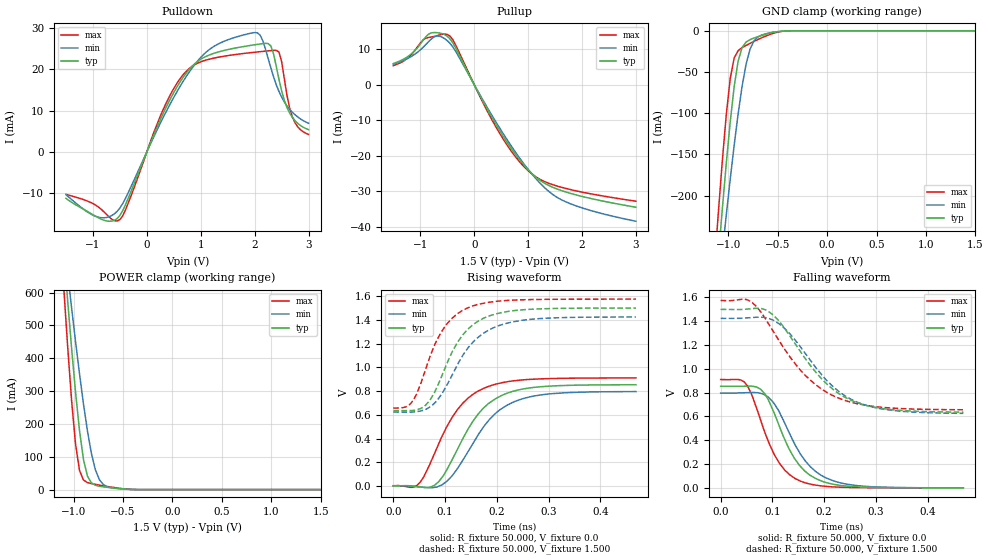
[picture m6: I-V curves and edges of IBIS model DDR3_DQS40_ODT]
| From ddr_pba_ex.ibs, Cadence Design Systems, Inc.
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|   Model DDR3_DQS40_ODT
[Model]   DDR3_DQS40_ODT
Model_type I/O
Polarity   Non-Inverting
Enable   Active-High
Vinl   =   0.703V
Vinh   =   0.796V
C_comp   1.640pF   1.630pF   1.688pF
C_comp_pullup   0.471pF   0.511pF   0.476pF
C_comp_pulldown 1.168pF   1.119pF   1.211pF
[Model Spec]
Vinh   0.796V   NA   NA
Vinl   0.703V   NA   NA
Vmeas   0.750V   NA   NA
[Add Submodel]
|  Submodel_name   Mode
DDR3_DQS_ODT60   Non-Driving
[Temperature Range]   27.000   0.125k   -40.000
[Voltage Range]   1.500V   1.425V   1.575V
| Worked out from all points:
|   slope of the pulldown table from 0 to 0.225 V, typ, clamps not added: 31.8 ohm
|   slope of the pullup table from 0 to 0.225 V, typ, clamps not added: 34.8 ohm
|   GND clamp passes 1 mA (typ) near -0.50 V on its own axis
|   POWER clamp passes 1 mA (typ) near -0.45 V on its own axis
|   rising waveform, R_fixture 50.000, V_fixture 0.0: 20-80 % time 73ps typ, 78.2ps min, 70.9ps max; typ from 0 V to 0.853 V
|   rising waveform, R_fixture 50.000, V_fixture 1.500: 20-80 % time 63.7ps typ, 72.4ps min, 57.6ps max; typ from 0.635 V to 1.5 V
|   falling waveform, R_fixture 50.000, V_fixture 0.0: 20-80 % time 58.1ps typ, 64.5ps min, 53.2ps max; typ from 0.854 V to 0 V
|   falling waveform, R_fixture 50.000, V_fixture 1.500: 20-80 % time 97.1ps typ, 96.2ps min, 101ps max; typ from 1.5 V to 0.636 V
[Pulldown]
|Voltage   I(typ)   I(min)   I(max)
-1.5V     -11.24mA   -10.36mA   -10.27mA
-900mV    -15.94mA   -15.8mA    -13.32mA
-500mV    -15.38mA   -13.58mA   -16.39mA
250mV     7.818mA    6.93mA     8.666mA
600mV     16.62mA    15.5mA     17.43mA
1.1V      23.14mA    24.16mA    22.24mA
1.7V      25.29mA    27.98mA    23.68mA
2.1V      26.12mA    28.29mA    24.27mA
2.3V      25.65mA    20.33mA    24.52mA
2.45V     17.59mA    14.66mA    24.19mA
2.7V      8.354mA    9.586mA    8.44mA
3V        5.378mA    6.93mA     4.234mA
[Pullup]
|Voltage   I(typ)   I(min)   I(max)
-1.5V     5.907mA    5.675mA    5.311mA
-1.2V     8.216mA    7.612mA    7.902mA
-950mV    12.44mA    10.43mA    12.49mA
-800mV    14.52mA    12.76mA    13.36mA
-650mV    14.53mA    13.64mA    13.93mA
-500mV    13.59mA    12.36mA    14.09mA
-350mV    10.47mA    9.5mA      11.3mA
450mV     -12.4mA    -11.68mA   -13.13mA
1V        -23.97mA   -23.85mA   -24.24mA
1.35V     -28.14mA   -29.63mA   -27.57mA
1.65V     -29.98mA   -32.65mA   -29.03mA
3V        -34.52mA   -38.47mA   -32.82mA
[GND_clamp]
|Voltage   I(typ)   I(min)   I(max)
-1.5V     -902.4mA   -795.2mA   -923mA
-1.14V    -333.6mA   -361.2mA   -285.4mA
-1.1V     -273.5mA   -314.1mA   -219.4mA
-1.06V    -215.4mA   -267.9mA   -157.1mA
-1.02V    -160.2mA   -222.9mA   -101.2mA
-980mV    -109.7mA   -179.4mA   -57.37mA
-940mV    -66.97mA   -138.2mA   -32.78mA
-900mV    -36.37mA   -100.2mA   -23.99mA
-820mV    -13.67mA   -40.29mA   -17.69mA
-740mV    -8.766mA   -12.21mA   -12.83mA
-540mV    -1.803mA   -1.643mA   -2.86mA
1.5V      1.904nA    275.5nA    464.3pA
[POWER_clamp]
|Voltage   I(typ)   I(min)   I(max)
-1.5V     2.395A     1.917A     2.689A
-1.1V     728.2mA    767.9mA    617.4mA
-1.06V    575.5mA    659.2mA    435.4mA
-1.02V    430.1mA    553.1mA    270.8mA
-980mV    295.8mA    450.4mA    137.9mA
-940mV    179.3mA    352.3mA    58.02mA
-900mV    91.53mA    260.8mA    29.3mA
-860mV    41.11mA    178.7mA    21.47mA
-780mV    13.3mA     60.49mA    15.94mA
-740mV    10.3mA     30.45mA    13.76mA
-620mV    5.486mA    5.676mA    7.71mA
1.5V      -5.523nA   -199nA     -1.165nA
[Ramp]
| variable   typ   min   max
dV/dt_r 0.512/74.400p   0.478/80.454p   0.547/71.752p
dV/dt_f 0.519/99.358p   0.481/97.096p   0.552/0.102n
R_load = 50.000
| The next line is not an IBIS keyword
| [Initial Delay]   0.225ns   0.350ns   0.175ns
[Rising Waveform]
R_fixture= 50.000
V_fixture= 0.0
V_fixture_min= 0.0
V_fixture_max= 0.0
|time   V(typ)   V(min)   V(max)
0s        427.1uV    1.408mV    2.698mV
46ps      -3.782mV   -5.48mV    5.951mV
59ps      -11.88mV   -11.65mV   78.51mV
87ps      33.15mV    -3.69mV    349mV
113ps     214.4mV    82.09mV    573.8mV
133ps     388.4mV    207.7mV    691.8mV
179ps     675.7mV    524.2mV    831mV
214ps     771.7mV    665.3mV    874mV
262ps     825.6mV    749.5mV    898mV
469ps     853.4mV    795.9mV    910.7mV
[Rising Waveform]
R_fixture= 50.000
V_fixture= 1.500
V_fixture_min= 1.425
V_fixture_max= 1.575
|time   V(typ)   V(min)   V(max)
0s        634.5mV    623.6mV    656.4mV
33ps      635.4mV    622.4mV    692.7mV
45ps      641.6mV    626.3mV    774.2mV
62ps      679mV      644.7mV    978.8mV
82ps      810.6mV    708mV      1.21V
101ps     1.006V     829.9mV    1.351V
142ps     1.312V     1.15V      1.498V
184ps     1.432V     1.313V     1.548V
231ps     1.477V     1.383V     1.566V
469ps     1.5V       1.425V     1.575V
[Falling Waveform]
R_fixture= 50.000
V_fixture= 0.0
V_fixture_min= 0.0
V_fixture_max= 0.0
|time   V(typ)   V(min)   V(max)
0s        853.8mV    796.2mV    910.2mV
46ps      854.6mV    799.7mV    888.8mV
60ps      855.2mV    801.8mV    783.3mV
78ps      825.7mV    793.5mV    558.4mV
92ps      740.7mV    763.4mV    391mV
113ps     522.6mV    641.1mV    210mV
153ps     186mV      291.5mV    58.59mV
193ps     60.68mV    108.6mV    17.14mV
239ps     16.65mV    35.02mV    4.345mV
469ps     190.3uV    184.7uV    90.24uV
[Falling Waveform]
R_fixture= 50.000
V_fixture= 1.500
V_fixture_min= 1.425
V_fixture_max= 1.575
|time   V(typ)   V(min)   V(max)
0s        1.5V       1.425V     1.574V
53ps      1.503V     1.429V     1.578V
69ps      1.51V      1.434V     1.525V
93ps      1.481V     1.424V     1.376V
123ps     1.345V     1.342V     1.169V
163ps     1.09V      1.133V     947.2mV
223ps     808.5mV    829.2mV    763mV
259ps     723.1mV    729.4mV    711.6mV
300ps     675.5mV    672.6mV    682.1mV
469ps     636.2mV    626.1mV    656.3mV
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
